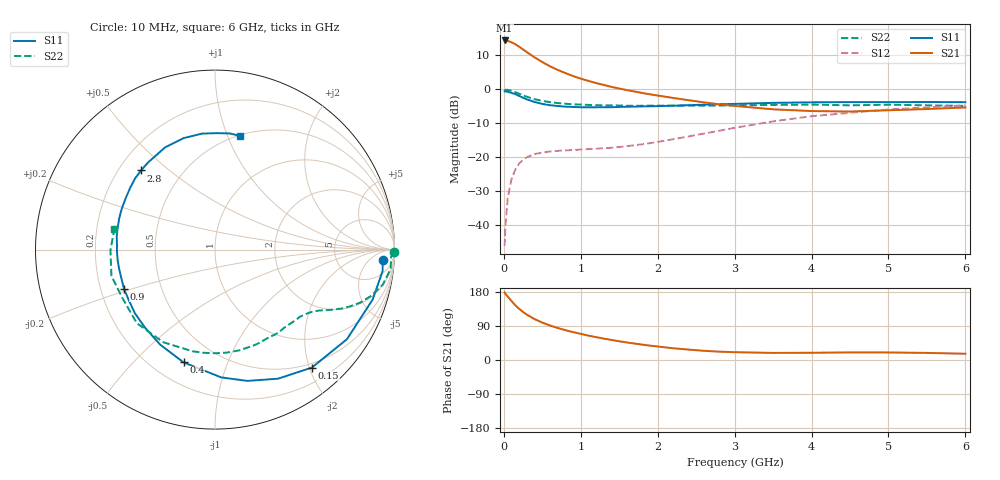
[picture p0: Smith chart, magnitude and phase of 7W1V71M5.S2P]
! Infineon Technologies  Discrete & RF Semiconductors
! BFS17W
! Si NPN RF Bipolar Junction Transistor in SOT323
! VCE = 1.75 V  IC = 1.5 mA
! Common Emitter S-Parameters:  August  1999
# GHz  S  MA  R  50
!  f  S11  S21  S12  S22
! GHz  MAG  ANG  MAG  ANG  MAG  ANG  MAG  ANG
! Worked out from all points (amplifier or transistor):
!   36 points, 10 MHz to 6 GHz, reference 50 ohm
!   highest |S21| = 14.4 dB at 10 MHz (marker M1)
!   |S21| within 3 dB of that: start of sweep to 271.7 MHz
!   unconditionally stable (mu >= 1): 874 MHz to end of sweep
!   at 250 MHz: K = 0.32, MSG = 16.3 dB, |S12| = -20.8 dB
!   at 1.4 GHz: K = 1.35, MAG = 5.4 dB, |S12| = -17.2 dB
!   at 6 GHz: K = 1.12, MAG = -2.4 dB, |S12| = -4.7 dB
!   S11 on the Smith chart (normalised r, x): 10 MHz: 17, -15; 150 MHz: 0.43, -2.04; 400 MHz: 0.32, -0.71; 900 MHz: 0.30, -0.19; 2.8 GHz: 0.29, +0.40; 6 GHz: 0.51, +1.11
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0.01  0.9359 -3.4  5.265 178.2  0.0049 83.8  0.9993 -0.8
0.02  0.9415 -7.3  5.26 175.0  0.0095 88.9  0.9815 -2.4
0.05  0.9213 -17.6  5.198 167.3  0.0248 81.0  0.9851 -6.2
0.1  0.8886 -34.2  4.946 155.6  0.0479 71.1  0.9553 -11.8
0.15  0.8505 -50.6  4.63 144.3  0.0664 62.2  0.9073 -16.5
0.2  0.8003 -64.0  4.262 134.9  0.0812 55.9  0.8622 -20.0
0.25  0.7533 -76.2  3.877 126.7  0.0916 49.9  0.816 -22.8
0.3  0.7129 -87.2  3.541 119.6  0.1003 46.2  0.7796 -24.9
0.4  0.6523 -105.6  2.966 107.8  0.1116 39.8  0.7176 -28.0
0.5  0.6112 -120.0  2.529 98.7  0.1171 36.0  0.678 -30.0
0.6  0.5844 -131.7  2.191 91.0  0.1217 34.1  0.6493 -31.9
0.7  0.5701 -141.5  1.94 84.5  0.1245 33.1  0.6302 -34.0
0.9  0.552 -156.8  1.574 73.6  0.1275 33.0  0.6029 -38.4
1.1  0.545 -169.1  1.335 64.3  0.1318 34.9  0.591 -43.4
1.3  0.5465 -179.1  1.163 56.4  0.1363 37.8  0.5812 -49.0
1.6  0.5561 168.7  0.976 46.2  0.1457 43.0  0.5751 -57.6
2.2  0.5746 149.7  0.749 31.0  0.1845 53.3  0.5773 -76.4
2.8  0.6034 133.0  0.604 22.0  0.246 57.2  0.5784 -96.3
3.5  0.6339 116.0  0.509 18.7  0.3383 54.4  0.5912 -119.2
4.5  0.6503 96.3  0.472 20.0  0.4525 42.8  0.5821 -152.4
5.5  0.6524 82.7  0.514 18.7  0.5435 30.9  0.5825 -179.7
6  0.6485 77.6  0.542 16.5  0.5788 25.2  0.5722 168.3
